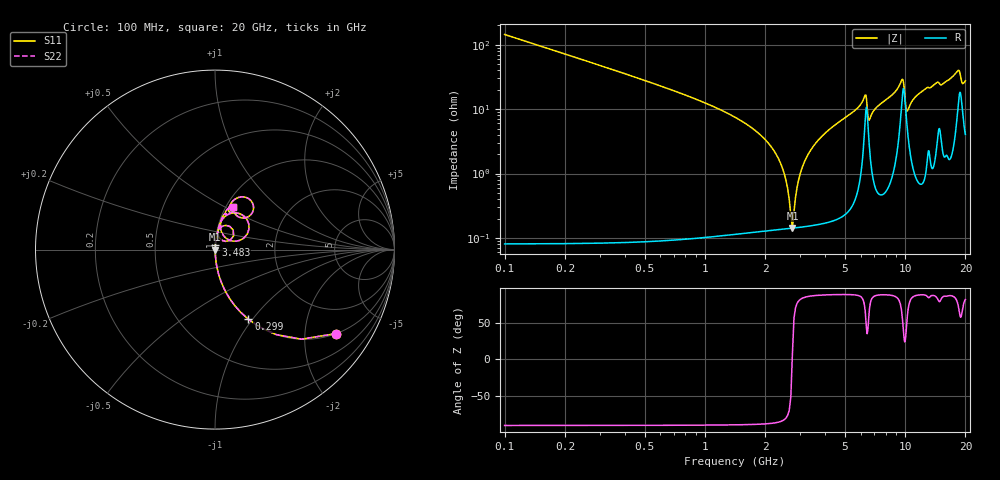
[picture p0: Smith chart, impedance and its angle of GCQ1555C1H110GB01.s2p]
!Murata Part Number: GCQ1555C1H110GB01
!These Parameters are Measured in Series Mode Connection
!Data Generated on Mar 13, 2026
!  o--ll--o
!Port1  Port2
!  o------o
!Operation Temp=25[degC], DC Bias Voltage=0[V]
!Freq. Start=100[MHz] Stop=20[GHz] 401[Steps]
# Hz S RI R 50
!Freq.(Hz) S11(Real) S11(Imag) S21(Real) S21(Imag) S12(Real) S12(Imag) S22(Real) S22(Imag)
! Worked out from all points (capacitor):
!   401 points, 100 MHz to 20 GHz, reference 50 ohm
!   read as one part in series: C = 11 pF near 199.5 MHz
!   lowest |Z| = 143 mohm at 2.737 GHz (marker M1)
!   series resonance near 2.732 GHz, so ESL is about 310 pH
!   S11 on the Smith chart (normalised r, x): 100 MHz: 1.00, -2.89; 299 MHz: 1.00, -0.96; 3.483 GHz: 1.00, +0.05; 20 GHz: 1.08, +0.55
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1e8  0.6761 -0.4677  0.3239 0.4677  0.3239 0.4677  0.6761 -0.4677
2.99e8  0.1865 -0.3886  0.8135 0.3886  0.8135 0.3886  0.1865 -0.3886
8.96e8  0.0213 -0.1409  0.9787 0.1409  0.9787 0.1409  0.0213 -0.1409
2.1895e9  0.00187 -0.0237  0.9981 0.0237  0.9981 0.0237  0.00187 -0.0237
2.43825e9  0.00151 -0.0121  0.9985 0.0121  0.9985 0.0121  0.00151 -0.0121
2.73675e9  0.00142 0.000187  0.9986 -0.000187  0.9986 -0.000187  0.00142 0.000187
3.03525e9  0.0016 0.0113  0.9984 -0.0113  0.9984 -0.0113  0.0016 0.0113
3.43325e9  0.00217 0.0248  0.9978 -0.0248  0.9978 -0.0248  0.00217 0.0248
3.483e9  0.00226 0.0264  0.9977 -0.0264  0.9977 -0.0264  0.00226 0.0264
6.269e9  0.0621 0.1346  0.9379 -0.1346  0.9379 -0.1346  0.0621 0.1346
6.5675e9  0.0414 0.0505  0.9586 -0.0505  0.9586 -0.0505  0.0414 0.0505
6.7665e9  0.019 0.0764  0.981 -0.0764  0.981 -0.0764  0.019 0.0764
9.60225e9  0.1473 0.1959  0.8527 -0.1959  0.8527 -0.1959  0.1473 0.1959
9.80125e9  0.1891 0.1138  0.8109 -0.1138  0.8109 -0.1138  0.1891 0.1138
1.005e10  0.099 0.0474  0.901 -0.0474  0.901 -0.0474  0.099 0.0474
1.0249e10  0.0534 0.0711  0.9466 -0.0711  0.9466 -0.0711  0.0534 0.0711
1.13435e10  0.0322 0.152  0.9678 -0.152  0.9678 -0.152  0.0322 0.152
1.338325e10  0.0573 0.2001  0.9427 -0.2001  0.9427 -0.2001  0.0573 0.2001
1.67165e10  0.0919 0.262  0.9081 -0.262  0.9081 -0.262  0.0919 0.262
1.865675e10  0.2148 0.2361  0.7852 -0.2361  0.7852 -0.2361  0.2148 0.2361
1.925375e10  0.1363 0.18  0.8637 -0.18  0.8637 -0.18  0.1363 0.18
2e10  0.1006 0.2357  0.8994 -0.2357  0.8994 -0.2357  0.1006 0.2357
